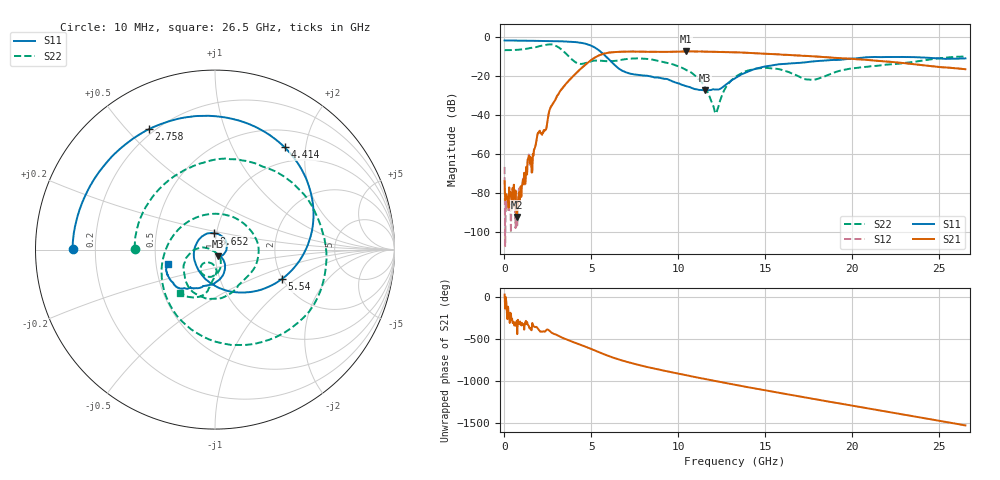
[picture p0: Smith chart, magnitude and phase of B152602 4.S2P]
!  2-Port S-parameters saved by WinCal
! VAR MeasName=S-Parameters (CALIBRATED_DATA) read from VNA (N5242A)
! VAR MeasDate=2016-1-5 16:25:57
! VAR NAME=B152602 4
! VAR FILENAME=B152602 4.S2P
! VAR DATE=2016-1-5 16:25:57
! VAR PHYS_PORTS=1,2
# Hz S DB R 50
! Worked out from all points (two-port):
!   801 points, 10 MHz to 26.5 GHz, reference 50 ohm
!   highest |S21| = -7.58 dB at 10.44 GHz (marker M1); lowest = -92.2 dB at 705.4 MHz (marker M2)
!   |S21| within 3 dB of the highest: 5.229 GHz to 18.52 GHz (13.29 GHz wide, 112 % of centre)
!   lowest |S11| = -27.5 dB at 11.53 GHz (marker M3), VSWR 1.09, Z = 51.7 - j3.97 ohm
!   |S11| at or under -10 dB: 5.814 GHz to end of sweep
!   |S22| runs from -39.2 to -4.0 dB; largest |S21 - S12| = 0.0033
!   S11 on the Smith chart (normalised r, x): 10 MHz: 0.11, +0.00; 2.758 GHz: 0.18, +0.58; 4.414 GHz: 0.75, +1.63; 5.54 GHz: 1.98, -0.78; 8.652 GHz: 0.98, +0.18; 26.5 GHz: 0.58, -0.10
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1e7  -2.00 179.8  -73.89 32.2  -66.63 -21.6  -6.96 179.3
1.755625e8  -2.02 176.4  -81.97 98.6  -83.13 103.9  -6.95 169.2
7.053625e8  -2.07 165.5  -92.16 78.4  -81.79 50.1  -6.81 136.5
1.5994e9  -2.19 146.9  -68.58 53.3  -69.50 53.0  -5.70 75.8
1.8643e9  -2.22 141.0  -52.13 1.5  -51.95 0.9  -5.29 55.3
2.294762e9  -2.27 130.9  -48.25 -50.2  -48.33 -50.7  -4.44 16.0
2.758338e9  -2.32 118.9  -34.69 -68.5  -34.67 -68.7  -4.13 -37.7
3.519925e9  -2.51 95.1  -24.36 -139.5  -24.38 -139.5  -8.55 -137.7
4.413962e9  -3.23 55.8  -16.26 149.2  -16.27 149.3  -13.99 88.6
4.447075e9  -3.28 54.0  -16.00 146.6  -16.01 146.8  -13.98 83.8
5.539788e9  -7.82 -23.8  -9.26 55.4  -9.25 55.5  -12.32 -25.6
6.566275e9  -16.32 -122.9  -7.81 -21.8  -7.80 -21.9  -12.12 -62.3
8.652362e9  -20.92 92.9  -7.82 -133.1  -7.82 -133.1  -12.08 -128.5
8.851038e9  -20.99 82.0  -7.84 -141.9  -7.84 -142.0  -12.47 -133.8
1.044044e10  -25.31 -31.9  -7.58 149.8  -7.58 150.0  -17.03 -171.3
1.153315e10  -27.48 -65.0  -7.67 104.1  -7.68 104.1  -26.11 169.3
1.216229e10  -27.04 -64.2  -7.80 79.1  -7.81 79.1  -39.21 -114.5
1.3255e10  -21.34 -53.2  -8.05 35.8  -8.05 35.7  -20.76 -69.3
1.570532e10  -14.26 -94.0  -9.09 -57.4  -9.08 -57.5  -16.55 -121.5
1.769208e10  -12.76 -111.9  -10.07 -130.3  -10.03 -130.3  -22.17 -107.4
2.209604e10  -10.45 -144.8  -12.86 70.7  -12.81 70.4  -14.30 -97.2
2.65e10  -11.16 -162.9  -16.70 -89.8  -16.70 -90.1  -10.23 -128.9
